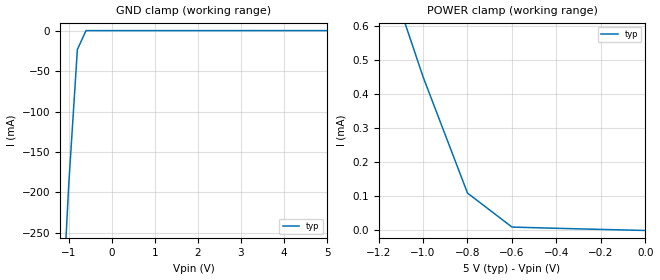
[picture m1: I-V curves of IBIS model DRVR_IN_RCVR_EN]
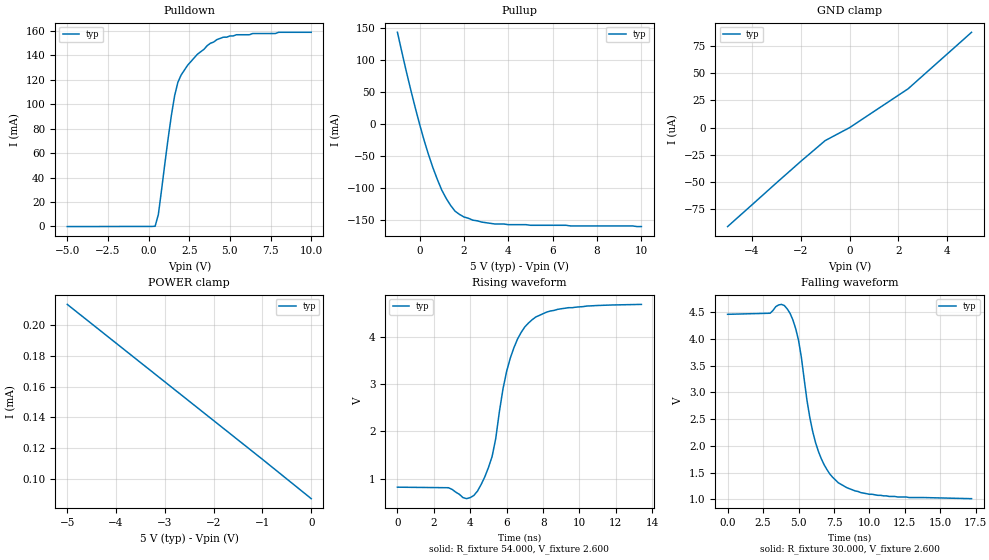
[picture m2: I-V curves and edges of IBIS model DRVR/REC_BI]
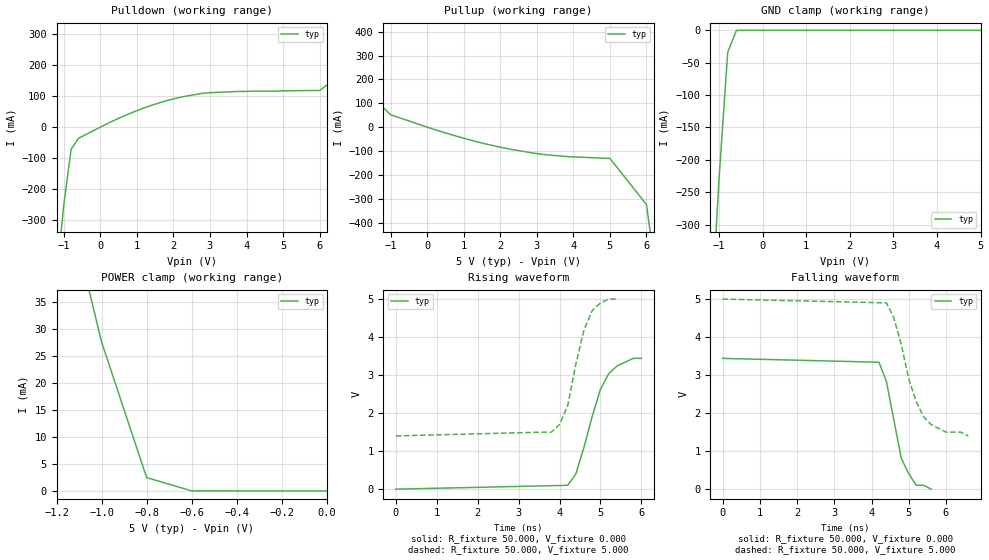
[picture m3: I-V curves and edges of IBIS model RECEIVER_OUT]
|   Texas Instruments Incorporated
|   Data Transmissions Products
|   IBIS Model for SN65HVD05
|   8D SOIC Package
[IBIS Ver]   3.2
[Comment char]   |_char
[File name]   hvd05.ibs
[File Rev]   1.1
[Date]   11Apr07
[Source]   File originated at Texas Instruments Incorporated.
   Data Transmission Products Group.
[Notes]
[Disclaimer]
(C) Copyright Texas Instruments Incorporated 2002
   All rights reserved
  Texas Instruments Incorporated hereby grants 1the user of this IBIS
model a non-exclusive, nontransferable license to use this IBIS model
under the following terms.  Before using this IBIS model, the user
should read this license.  If the user does not accept these terms,
the IBIS model should be returned to Texas Instruments within 30 days.
  The user is granted this license only to use the IBIS model and
is not granted rights to sell, load, rent, lease or license the IBIS
model in whole or in part, or in modified form to anyone other than
user.  User may modify the IBIS model to suit its specific applications
but rights to derivative works and such modifications shall belong to
Texas Instruments.
  This IBIS model is provided on an "AS IS" basis and Texas Instruments
makes absolutely no warranty with respect to the information contained
herein.  TEXAS INSTRUMENTS DISCLAIMS AND CUSTOMER WAIVES ALL WARRANTIES,
EXPRESS OR IMPLIED, INCLUDING WARRANTIES OF MERCHANTABILITY OR FITNESS
FOR A PARTICULAR PURPOSE. The entire risk as to quality and performance
is with the Customer. ACCORDINGLY, IN NO EVENT SHALL THE COMPANY BE LIABLE
FOR ANY DAMAGES, WHETHER IN CONTRACT OR TORT,INCLUDING ANY LOST PROFITS
OR OTHER INCIDENTAL, CONSEQUENTIAL, EXEMPLARY, OR PUNITIVE DAMAGES ARISING
OUT OF THE USE OR APPLICATION OF THE IBIS model provided in this package.
Further, Texas Instruments reserves the right to discontinue or make changes
without notice to any product herein to improve reliability, function, or
design. Texas Instruments does not convey any license under patent rights
or any other intellectual property rights, including those of third parties.
Contact Texas Instruments at ATTN:DATA TRANSMISSIONS
[Copyright]   Copyright 2002, Texas Instruments, All Rights Reserved
[Component]   HVD05D
[Manufacturer]  Texas Instruments Incorporated
[Package]
|   typ   min   max
R_pkg   0.036   0.033   0.039
L_pkg   3.340nH   2.445nH   4.233nH
C_pkg   0.470pF   0.308pF   0.631pF
[Pin]   signal_name   model_name   R_pin   L_pin   C_pin
1   R   RECEIVER_OUT   0.034   4.233n   0.630p
2   RE   DRVR_IN_RCVR_EN   0.038   2.445n   0.309p
3   DE   DRIVER_EN   0.039   2.448n   0.309p
4   D   DRVR_IN_RCVR_EN   0.033   4.231n   0.631p
5   GND   GND   0.033   4.230n   0.630p
6   A   DRVR/REC_BI   0.039   2.450n   0.308p
7   B   DRVR/REC_BI   0.039   2.448n   0.309p
8   VCC   POWER   0.033   4.231n   0.630p
[Diff_pin]   inv_pin   vdiff   tdelay_typ   tdelay_min   tdelay_max
| The 'A' pin is Diff_pin and the 'B' pin is the inv_pin
6   7   0.200   0 0 0
| Models and submodels in the file (4): DRVR_IN_RCVR_EN (Input), DRIVER_EN (Input), DRVR/REC_BI (I/O), RECEIVER_OUT (3-state)
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|   Driver Input / Receiver Enable Model
[Model]   DRVR_IN_RCVR_EN
Model_type   Input
|Signals   D,RE
Vinh = 2.0
Vinl = 0.8
|   typ   min   max
C_comp   1.0pF   NA   NA
|   typ   min   max
[Temperature Range]   25.0   NA   NA
[Voltage range]   5.0V   4.5V   5.5V
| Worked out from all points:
|   GND clamp passes 1 mA (typ) near -0.61 V on its own axis
|   POWER clamp passes 1 mA (typ) near -1.28 V on its own axis
[GND_clamp]
|   Voltage   I(typ)   I(min)   I(max)
-5V       -4.2A      NA         NA
-4V       -3.22A     NA         NA
-3V       -2.23A     NA         NA
-2V       -1.22A     NA         NA
-1V       -190mA     NA         NA
-800mV    -23.4mA    NA         NA
-600mV    -55.7uA    NA         NA
-400mV    -27.7uA    NA         NA
-200mV    -27.7uA    NA         NA
0V        -27.6uA    NA         NA
2.4V      -25.3uA    NA         NA
5V        12pA       NA         NA
[Power_clamp]
| Note that the[POWER_clamp]voltage table is referenced to Vcc
| and is calculated using Vtable=Vcc - Vmeasured.
|   Voltage   I(typ)   I(min)   I(max)
-5V       8.78mA     NA         NA
-1.2V     841uA      NA         NA
-1V       452uA      NA         NA
-800mV    110uA      NA         NA
-600mV    10uA       NA         NA
0V        12pA       NA         NA
|   Driver Output / Receiver Input Model
[Model]   DRVR/REC_BI
Model_type   I/O
| Signals   A,B
Vinl = 4.3V
Vinh = 1.0V
Vmeas = 2.6V   |Reference voltage for timing measurements
Cref = 50pF   |Timing specification test load capacitance value
Rref = 54   |Note: 54 Ohm load; single ended configuration
|   Timing specification test load voltage
| variable   typ   min   max
C_comp   32pF   26pF   38pF
|   typ   min   max
[Temperature Range]   25.0   NA   NA
[Voltage range]   5.0V   4.5V   5.5V
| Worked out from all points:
|   slope of the pulldown table from 0 to 0.75 V, typ, clamps not added: 29.9 ohm
|   slope of the pullup table from 0 to 0.75 V, typ, clamps not added: 9.17 ohm
|   rising waveform, R_fixture 54.000, V_fixture 2.600: 20-80 % time 1.29ns typ, NA min, NA max; typ from 0.826 V to 4.68 V
|   falling waveform, R_fixture 30.000, V_fixture 2.600: 20-80 % time 1.58ns typ, NA min, NA max; typ from 4.46 V to 1.01 V
[Pulldown]
|   Voltage   I(typ)   I(min)   I(max)
-5V       -152uA     NA         NA
400mV     75.4uA     NA         NA
600mV     9.68mA     NA         NA
1.2V      71.9mA     NA         NA
1.4V      90.8mA     NA         NA
1.6V      107mA      NA         NA
1.8V      118mA      NA         NA
2.4V      132mA      NA         NA
3.6V      148mA      NA         NA
4.6V      155mA      NA         NA
6.4V      158mA      NA         NA
10V       159mA      NA         NA
[Pullup]
|   Voltage   I(typ)   I(min)   I(max)
| Note that the[Pullup]voltage table is referenced to Vcc
| and is calculated using Vtable=Vcc - Vmeasured.
-1V       144mA      NA         NA
-600mV    82.8mA     NA         NA
-200mV    26.4mA     NA         NA
400mV     -47.3mA    NA         NA
600mV     -67.9mA    NA         NA
1V        -103mA     NA         NA
1.2V      -116mA     NA         NA
1.6V      -136mA     NA         NA
2V        -145mA     NA         NA
2.4V      -150mA     NA         NA
3.4V      -156mA     NA         NA
10V       -160mA     NA         NA
[GND_clamp]
|   Voltage   I(typ)   I(min)   I(max)
| Outputs in High Impedance (off)
-5V       -90.9uA    NA         NA
-4V       -70.9uA    NA         NA
-3V       -50.8uA    NA         NA
-2V       -31uA      NA         NA
-1V       -11.9uA    NA         NA
0V        -612pA     NA         NA
2.4V      35.7uA     NA         NA
5V        87.6uA     NA         NA
[POWER_clamp]
|   Voltage   I(typ)   I(min)   I(max)
| Note that the [POWER_clamp] voltage table is referenced to Vcc
| and is calculated using Vtable = Vcc - Vmeasured.
| Outputs in Tri-state.
-5V       213uA      NA         NA
-4V       188uA      NA         NA
-3V       163uA      NA         NA
-2V       138uA      NA         NA
-1V       113uA      NA         NA
0V        87.6uA     NA         NA
[Ramp]
|   typ   min   max
dV/dt_r   2.00/1.3ns   NA   NA
dV/dt_f   2.01/2.5ns   NA   NA
R_load = 54ohm | Note: The measurement is on a single-ended configuration
|   with 54ohm line-to-line.
[Rising Waveform]
R_fixture = 54.000
V_fixture = 2.600
C_fixture = 0.000
L_fixture = 0.000
|  time   V(typ)   V(min)   V(max)
0s        825.9mV    NA         NA
2.8ns     814.4mV    NA         NA
3.8ns     583.8mV    NA         NA
4.4ns     745.2mV    NA         NA
5.2ns     1.472V     NA         NA
5.8ns     2.901V     NA         NA
6.2ns     3.547V     NA         NA
6.8ns     4.089V     NA         NA
7.6ns     4.412V     NA         NA
13.4ns    4.677V     NA         NA
[Falling Waveform]
R_fixture = 30.000
V_fixture = 2.600
C_fixture = 0.000
L_fixture = 0.000
|  time   V(typ)   V(min)   V(max)
0s        4.457V     NA         NA
3.8ns     4.642V     NA         NA
4.2ns     4.56V      NA         NA
5ns       3.974V     NA         NA
5.6ns     2.843V     NA         NA
6.2ns     2.062V     NA         NA
6.8ns     1.651V     NA         NA
7.8ns     1.312V     NA         NA
10.6ns    1.076V     NA         NA
17.2ns    1.014V     NA         NA
[Model]   RECEIVER_OUT
Model_type   3-state
| Signals   R
Vmeas = 1.5V   |Reference voltage for timing measurements
Cref = 15pF   |Timing specification test load capacitance value
Vref = 0   |Timing specification test load voltage; GND
| variable   typ   min   max
C_comp   1.0pF   NA   NA
|   typ   min   max
[Temperature Range]   25.0   NA   NA
[Voltage range]   5.0V   4.5V   5.5V
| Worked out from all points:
|   slope of the pulldown table from 0 to 0.75 V, typ, clamps not added: 18.2 ohm
|   slope of the pullup table from 0 to 0.75 V, typ, clamps not added: 21 ohm
|   GND clamp passes 1 mA (typ) near -0.61 V on its own axis
|   POWER clamp passes 1 mA (typ) near -0.68 V on its own axis
|   rising waveform, R_fixture 50.000, V_fixture 0.000: 20-80 % time 580ps typ, NA min, NA max; typ from 0 V to 3.44 V
|   falling waveform, R_fixture 50.000, V_fixture 0.000: 20-80 % time 444ps typ, NA min, NA max; typ from 3.44 V to 0 V
|   rising waveform, R_fixture 50.000, V_fixture 5.000: 20-80 % time 464ps typ, NA min, NA max; typ from 1.4 V to 5 V
|   falling waveform, R_fixture 50.000, V_fixture 5.000: 20-80 % time 627ps typ, NA min, NA max; typ from 5 V to 1.4 V
[Pulldown]
|   Voltage   I(typ)   I(min)   I(max)
-5V       -4.95A     NA         NA
-2V       -1.44A     NA         NA
-1V       -249mA     NA         NA
-800mV    -70.9mA    NA         NA
-600mV    -35.9mA    NA         NA
400mV     23mA       NA         NA
1.6V      77.8mA     NA         NA
2.8V      109mA      NA         NA
6V        118mA      NA         NA
7V        204mA      NA         NA
8V        381mA      NA         NA
10V       741mA      NA         NA
[Pullup]
|   Voltage   I(typ)   I(min)   I(max)
| Note that the[Pullup]voltage table is referenced to Vcc
| and is calculated using Vtable=Vcc - Vmeasured.
-5V       741mA      NA         NA
-4V       560mA      NA         NA
-3V       380mA      NA         NA
-2V       202mA      NA         NA
-1V       51.7mA     NA         NA
800mV     -37.9mA    NA         NA
2.2V      -90.4mA    NA         NA
3.2V      -115mA     NA         NA
5V        -131mA     NA         NA
6V        -324mA     NA         NA
7V        -1.44A     NA         NA
10V       -4.95A     NA         NA
[GND_clamp]
|   Voltage   I(typ)   I(min)   I(max)
| Outputs in High Impedance (off)
-5V       -4.95A     NA         NA
-4V       -3.79A     NA         NA
-3V       -2.62A     NA         NA
-2V       -1.43A     NA         NA
-1V       -230mA     NA         NA
-800mV    -33.8mA    NA         NA
-600mV    -137uA     NA         NA
-400mV    -384nA     NA         NA
-200mV    -485pA     NA         NA
0V        -60pA      NA         NA
2V        -9.43pA    NA         NA
5V        66.4pA     NA         NA
[POWER_clamp]
|   Voltage   I(typ)   I(min)   I(max)
| Note that the [POWER_clamp] voltage table is referenced to Vcc
| and is calculated using Vtable = Vcc - Vmeasured.
| Outputs in Tri-state.
-5V       741mA      NA         NA
-4V       560mA      NA         NA
-3V       380mA      NA         NA
-2V       200mA      NA         NA
-1V       27.6mA     NA         NA
-800mV    2.47mA     NA         NA
-600mV    1.82uA     NA         NA
-400mV    894pA      NA         NA
-200mV    71.9pA     NA         NA
0V        66.4pA     NA         NA
[Ramp]
|   typ   min   max
dV/dt_r   4.10V/2.16ns   NA   NA
dV/dt_f   3.86V/3.15ns   NA   NA
R_load = 50
[Rising Waveform]
R_fixture = 50.000
V_fixture = 0.000
C_fixture = 0.000
L_fixture = 0.000
|  time   V(typ)   V(min)   V(max)
0s        2.127nV    NA         NA
4.2ns     101.2mV    NA         NA
4.4ns     404.7mV    NA         NA
4.6ns     1.113V     NA         NA
4.8ns     1.922V     NA         NA
5ns       2.631V     NA         NA
5.2ns     3.035V     NA         NA
5.4ns     3.238V     NA         NA
5.8ns     3.44V      NA         NA
6ns       3.44V      NA         NA
[Falling Waveform]
R_fixture = 50.000
V_fixture = 0.000
C_fixture = 0.000
L_fixture = 0.000
|  time   V(typ)   V(min)   V(max)
0s        3.44V      NA         NA
4.2ns     3.339V     NA         NA
4.4ns     2.833V     NA         NA
4.6ns     1.821V     NA         NA
4.8ns     809.4mV    NA         NA
5ns       404.7mV    NA         NA
5.2ns     101.2mV    NA         NA
5.4ns     101.2mV    NA         NA
5.6ns     2.127nV    NA         NA
[Rising Waveform]
R_fixture = 50.000
V_fixture = 5.000
C_fixture = 0.000
L_fixture = 0.000
|  time   V(typ)   V(min)   V(max)
0s        1.4V       NA         NA
3.8ns     1.5V       NA         NA
4ns       1.7V       NA         NA
4.2ns     2.2V       NA         NA
4.4ns     3.3V       NA         NA
4.6ns     4.2V       NA         NA
4.8ns     4.7V       NA         NA
5ns       4.9V       NA         NA
5.2ns     5V         NA         NA
5.4ns     5V         NA         NA
[Falling Waveform]
R_fixture = 50.000
V_fixture = 5.000
C_fixture = 0.000
L_fixture = 0.000
|  time   V(typ)   V(min)   V(max)
0s        5V         NA         NA
4.4ns     4.9V       NA         NA
4.6ns     4.5V       NA         NA
4.8ns     3.8V       NA         NA
5ns       2.9V       NA         NA
5.2ns     2.3V       NA         NA
5.4ns     1.9V       NA         NA
5.6ns     1.7V       NA         NA
6ns       1.5V       NA         NA
6.6ns     1.4V       NA         NA
